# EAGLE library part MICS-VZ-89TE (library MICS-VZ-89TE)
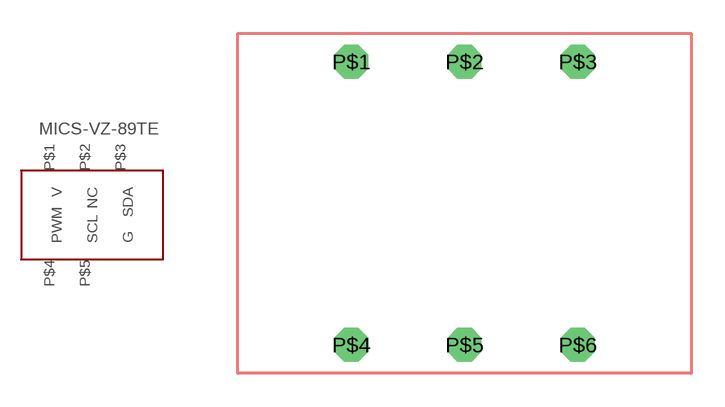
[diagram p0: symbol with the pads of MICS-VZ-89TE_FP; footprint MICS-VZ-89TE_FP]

Designator prefix -

## MICS-VZ-89TE  [MICS-VZ-89TE_FP]
P$1  V
P$2  NC
P$3  SDA
P$4  PWM
P$5  SCL
P$6  G

## Footprint MICS-VZ-89TE_FP (pad centres in mm)
drill 1.016 octagon: P$1 0,0; P$2 5.08,0; P$3 10.16,0; P$4 0,-12.7; P$5 5.08,-12.7; P$6 10.16,-12.7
